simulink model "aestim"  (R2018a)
settings: Solver=VariableStepAuto  StartTime=0.0  StopTime=10.0  RelTol=1e-3
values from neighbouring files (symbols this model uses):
  d2r = 1/r2d    (= 0.0174532925199)    [init.m]

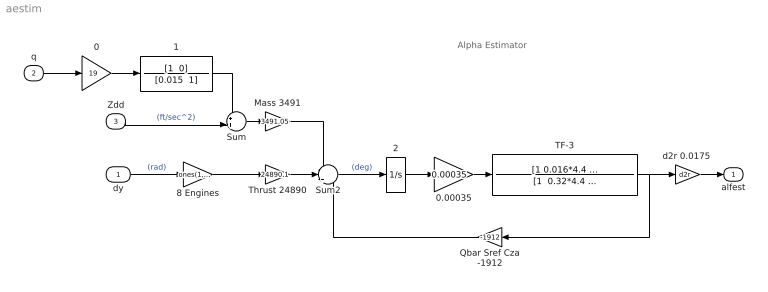
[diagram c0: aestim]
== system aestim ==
  note: Alpha Estimator
  dy : Inport
  q : Inport  Port=2
  Zdd : Inport  Port=3
  0 : Gain  Gain=19
  0.00035 : Gain  Gain=0.00035
  1 : TransferFcn  Numerator="[1  0]"  Denominator="[0.015  1]"
  2 : Integrator
  8 Engines : Gain  Gain=ones(1,8)  Multiplication=Matrix(K*u) (u vector)
  Mass 3491 : Gain  Gain=3491.05
  Qbar Sref Cza -1912 : Gain  Gain=-1912
  Sum : Sum  Inputs=++|
  Sum2 : Sum  Inputs=--+
  TF-3 : TransferFcn  Numerator="[1 0.016*4.4  4.38^2]"  Denominator="[1  0.32*4.4  4.38^2]"
  Thrust 24890 : Gain  Gain=24890.1
  "d2r 0.0175 " : Gain  Gain=d2r
  alfest : Outport
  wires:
  q/1 -> 0/1
  Sum2/1 -> 2/1  "(deg)"
  Qbar Sref Cza -1912/1 -> Sum2/3
  TF-3/1 -> "d2r 0.0175 "/1, Qbar Sref Cza -1912/1
  Thrust 24890/1 -> Sum2/2
  "d2r 0.0175 "/1 -> alfest/1
  Mass 3491/1 -> Sum2/1
  8 Engines/1 -> Thrust 24890/1
  Sum/1 -> Mass 3491/1
  2/1 -> 8 Engines/1  "(rad)"
  Zdd/1 -> Sum/2  "(ft/sec^2)"
  2/1 -> 0.00035/1
  0.00035/1 -> TF-3/1
  0/1 -> 1/1
  1/1 -> Sum/1
